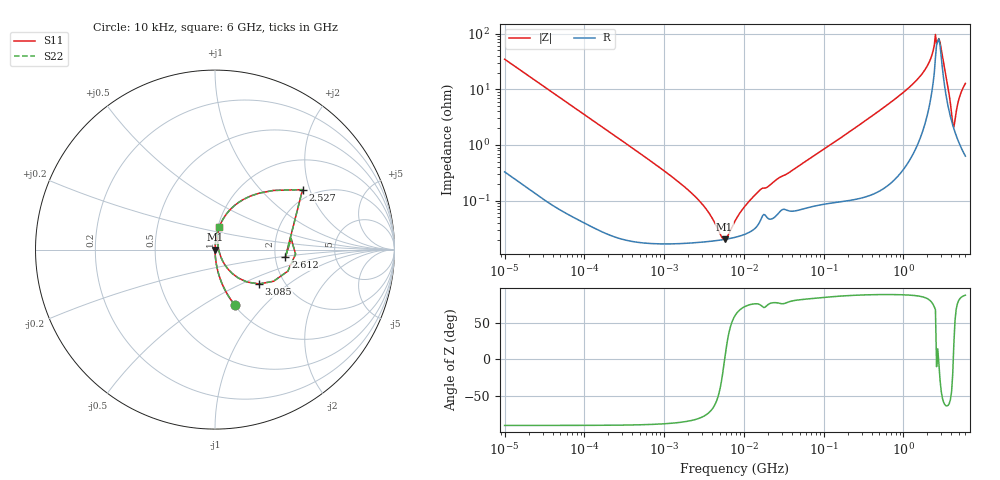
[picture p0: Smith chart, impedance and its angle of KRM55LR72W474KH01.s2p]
!Murata Part Number: KRM55LR72W474KH01
!These Parameters are Measured in Series Mode Connection
!Data Generated on Jan 08, 2026
!  o--ll--o
!Port1  Port2
!  o------o
!Operation Temp=25[degC], DC Bias Voltage=0[V]
!Freq. Start=10[kHz] Stop=6[GHz] 401[Steps]
# Hz S RI R 50
!Freq.(Hz) S11(Real) S11(Imag) S21(Real) S21(Imag) S12(Real) S12(Imag) S22(Real) S22(Imag)
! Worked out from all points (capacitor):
!   401 points, 10 kHz to 6 GHz, reference 50 ohm
!   read as one part in series: C = 457 nF near 10.69 kHz
!   lowest |Z| = 20.1 mohm at 5.742 MHz (marker M1)
!   series resonance near 5.741 MHz, so ESL is about 1.7 nH
!   S11 on the Smith chart (normalised r, x): 10 kHz: 1.01, -0.70; 2.527 GHz: 1.74, +1.79; 2.612 GHz: 2.28, -0.22; 3.085 GHz: 1.49, -0.63; 6 GHz: 1.01, +0.26
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10000  0.1102 -0.3085  0.8898 0.3085  0.8898 0.3085  0.1102 -0.3085
28042  0.0164 -0.1226  0.9836 0.1226  0.9836 0.1226  0.0164 -0.1226
92862  0.00185 -0.0378  0.9982 0.0378  0.9982 0.0378  0.00185 -0.0378
862344  0.000183 -0.004  0.9998 0.004  0.9998 0.004  0.000183 -0.004
2762288  0.000179 -0.000976  0.9998 0.000976  0.9998 0.000976  0.000179 -0.000976
5742053  0.000201 2e-07  0.9998 -2e-07  0.9998 -2e-07  0.000201 2e-07
7745967  0.000219 0.000369  0.9998 -0.000369  0.9998 -0.000369  0.000219 0.000369
1.610178e7  0.000439 0.00151  0.9996 -0.00151  0.9996 -0.00151  0.000439 0.00151
7.193098e7  0.000816 0.00602  0.9992 -0.00602  0.9992 -0.00602  0.000816 0.00602
6.67969e8  0.00505 0.0556  0.9949 -0.0556  0.9949 -0.0556  0.00505 0.0556
1.873109e9  0.0686 0.2043  0.9314 -0.2043  0.9314 -0.2043  0.0686 0.2043
2.139659e9  0.1302 0.262  0.8698 -0.262  0.8698 -0.262  0.1302 0.262
2.364181e9  0.2478 0.3149  0.7522 -0.3149  0.7522 -0.3149  0.2478 0.3149
2.526803e9  0.4878 0.3339  0.5122 -0.3339  0.5122 -0.3339  0.4878 0.3339
2.612262e9  0.3927 -0.0407  0.6073 0.0407  0.6073 0.0407  0.3927 -0.0407
2.791949e9  0.449 -0.0248  0.551 0.0248  0.551 0.0248  0.449 -0.0248
3.084918e9  0.245 -0.1914  0.755 0.1914  0.755 0.1914  0.245 -0.1914
3.523913e9  0.0717 -0.1078  0.9283 0.1078  0.9283 0.1078  0.0717 -0.1078
4.025378e9  0.0269 -0.0245  0.9731 0.0245  0.9731 0.0245  0.0269 -0.0245
4.302268e9  0.0192 0.00742  0.9808 -0.00742  0.9808 -0.00742  0.0192 0.00742
5.252544e9  0.016 0.0823  0.984 -0.0823  0.984 -0.0823  0.016 0.0823
6e9  0.022 0.1239  0.978 -0.1239  0.978 -0.1239  0.022 0.1239
